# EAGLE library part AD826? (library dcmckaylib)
High speed (50MHz) dual op-amp 15nV/Hz^(0.5) voltage noise, 1.5pA/Hz^(0.5) current noise 15nA offset current (10uA bias)
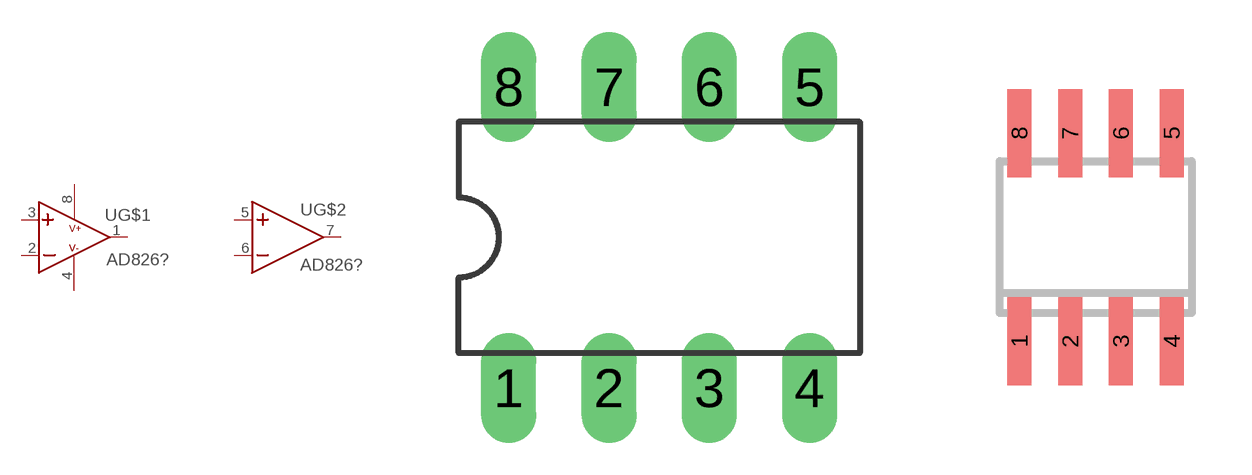
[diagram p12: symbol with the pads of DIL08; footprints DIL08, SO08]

Designator prefix U; gates G$1=OPAMP2 G$2=OPAMP

## AD826AN  [DIL08]
1  G$1:OUT  out
2  G$1:IN-  in
3  G$1:IN+  in
4  G$1:V-  pwr
5  G$2:IN+  in
6  G$2:IN-  in
7  G$2:OUT  out
8  G$1:V+  pwr

## AD826AR  [SO08]
Pads as for DIL08

## Footprint DIL08 (pad centres in mm)
Dual In Line Package
drill 0.889 long: 1 -3.81,-3.81; 2 -1.27,-3.81; 3 1.27,-3.81; 4 3.81,-3.81; 5 3.81,3.81; 6 1.27,3.81; 7 -1.27,3.81; 8 -3.81,3.81

## Footprint SO08 (pad centres in mm)
Small Outline Package 8 NS Package M08A
smd 0.6 x 2.2: 1 -1.905,-2.6; 2 -0.635,-2.6; 3 0.635,-2.6; 4 1.905,-2.6; 5 1.905,2.6; 6 0.635,2.6; 7 -0.635,2.6; 8 -1.905,2.6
